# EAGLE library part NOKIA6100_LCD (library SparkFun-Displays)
Nokia 6100 Color LCD Previously used in production. SparkFun Products: 128x128 Nokia Knock-Off (Retired) Color LCD SMD connector
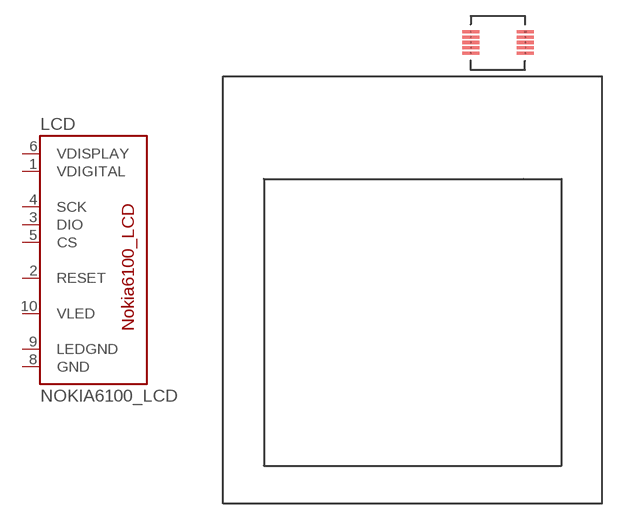
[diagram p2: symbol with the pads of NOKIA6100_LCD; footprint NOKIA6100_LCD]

Designator prefix LCD

## NOKIA6100_LCD (SF_ID: LCD-00570)  [NOKIA6100_LCD]
1  VDIGITAL
2  RESET
3  DIO
4  SCK
5  CS
6  VDISPLAY
8  GND
9  LEDGND
10  VLED

## Footprint NOKIA6100_LCD (pad centres in mm)
Nokia 6100 LED Shape and Connector For Nokia-type LCDs. Specifications: Pin count: 10 Pin pitch: " Area: Datasheet referenced for footprint: Example device(s): Retired Color LCD
smd 1.6 x 0.3: 1 24.255,44.311; 2 24.255,43.811; 3 24.255,43.311; 4 24.255,42.811; 5 24.255,42.311; 6 29.389,42.303; 7 29.389,42.803; 8 29.389,43.303; 9 29.389,43.803; 10 29.389,44.303

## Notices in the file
Licensing: Creative Commons ShareAlike 4.0 International - https://creativecommons.org/licenses/by-sa/4.0
